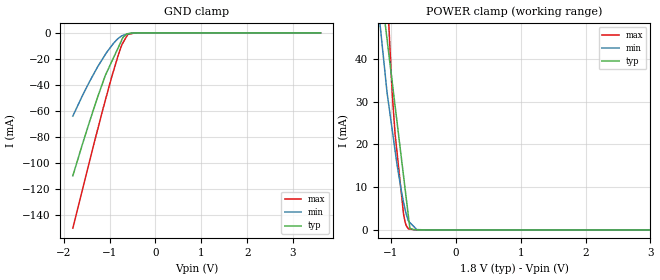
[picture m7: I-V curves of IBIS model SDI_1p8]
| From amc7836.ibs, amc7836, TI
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|   Model
[Model]   SDI_1p8
Model_type   Input
Vinl = 0.54
Vinh = 1.26
|   typ   min   max
C_comp   5.695pF   5.385pF   6.233pF
[Voltage Range]   1.8   1.79   1.81
[Temperature Range]   27   125   -40
[Power Clamp Reference]   1.8   1.79   1.81
[GND Clamp Reference]   0   0   0
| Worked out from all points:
|   GND clamp passes 1 mA (typ) near -0.62 V on its own axis
|   POWER clamp passes 1 mA (typ) near -0.71 V on its own axis
[GND Clamp]
|   Voltage   I(typ)   I(min)   I(max)
-1.8V     -109.7mA   -63.85mA   -149.9mA
-1.438V   -68.41mA   -37.54mA   -98.9mA
-1.255V   -48.81mA   -25.78mA   -73.56mA
-1.093V   -32.71mA   -16.67mA   -51.87mA
-909mV    -18.77mA   -7.811mA   -28.67mA
-763.2mV  -7.711mA   -2.96mA    -12.15mA
-730.8mV  -5.252mA   -2.235mA   -9.023mA
-709mV    -3.598mA   -1.957mA   -7.703mA
-660.6mV  -1.852mA   -1.338mA   -4.773mA
-601.2mV  -740.9uA   -579.4uA   -1.177mA
-433.8mV  -9.174uA   -52.99uA   -8.582uA
3.6V      0A         0A         0A
[POWER Clamp]
|   Voltage   I(typ)   I(min)   I(max)
-1.8V     276.3mA    209.7mA    333mA
-1.19V    75.32mA    51.29mA    99.5mA
-1.136V   60.53mA    43.32mA    80.04mA
-1.093V   48.7mA     36.94mA    66.58mA
-1.06V    44.63mA    32.16mA    56.49mA
-990mV    35.79mA    24.46mA    34.63mA
-936mV    29mA       18.54mA    22.39mA
-806.5mV  12.71mA    6.525mA    3.822mA
-730.8mV  3.186mA    2.086mA    250.9uA
-709mV    443.5uA    1.75mA     208.8uA
-649.8mV  51.12uA    837uA      94.37uA
3.6V      0A         0A         0A
